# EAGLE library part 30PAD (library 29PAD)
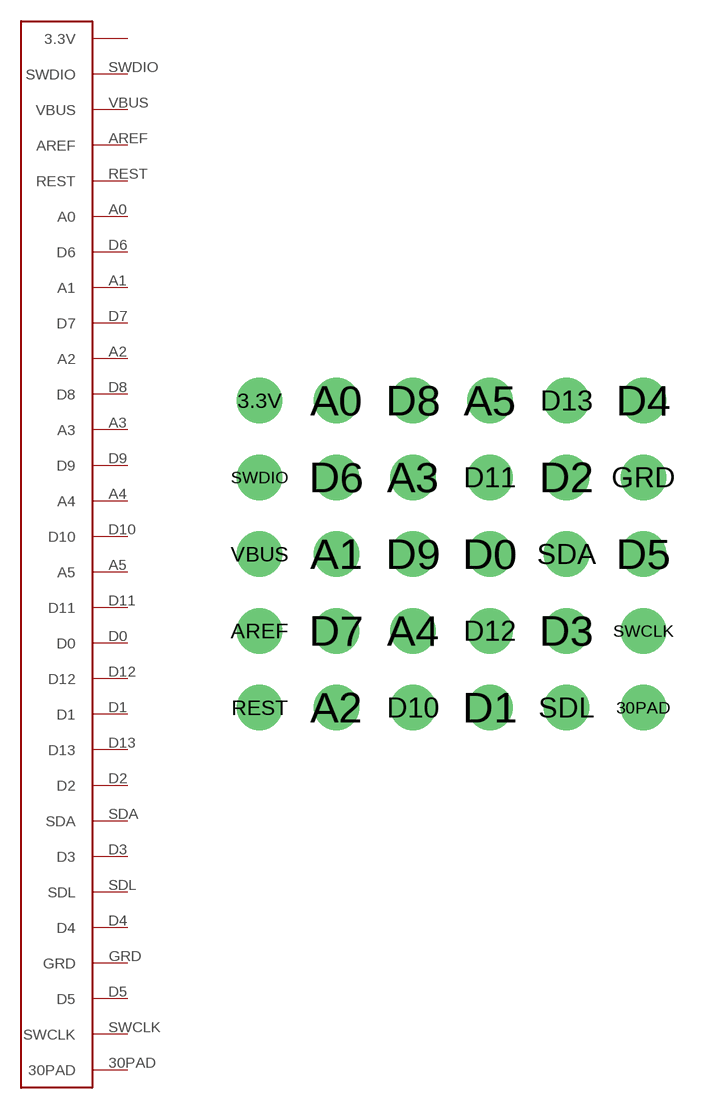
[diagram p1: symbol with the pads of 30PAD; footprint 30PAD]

Designator prefix -

## 30PAD  [30PAD]
3.3V  3.3V
30PAD  30PAD  nc
A0  A0
A1  A1
A2  A2
A3  A3
A4  A4
A5  A5
AREF  AREF
D0  D0
D1  D1
D2  D2
D3  D3
D4  D4
D5  D5
D6  D6
D7  D7
D8  D8
D9  D9
D10  D10
D11  D11
D12  D12
D13  D13
GRD  GRD
REST  REST
SDA  SDA
SDL  SDL
SWCLK  SWCLK
SWDIO  SWDIO
VBUS  VBUS

## Footprint 30PAD (pad centres in mm)
drill 1 pad 1.4: 3.3V -6.35,12.16; 30PAD 6.35,2; A0 -3.81,12.16; A1 -3.81,7.08; A2 -3.81,2; A3 -1.27,9.62; A4 -1.27,4.54; A5 1.27,12.16; AREF -6.35,4.54; D0 1.27,7.08; D1 1.27,2; D2 3.81,9.62; D3 3.81,4.54; D4 6.35,12.16; D5 6.35,7.08; D6 -3.81,9.62; D7 -3.81,4.54; D8 -1.27,12.16; D9 -1.27,7.08; D10 -1.27,2; D11 1.27,9.62; D12 1.27,4.54; D13 3.81,12.16; GRD 6.35,9.62; REST -6.35,2; SDA 3.81,7.08; SDL 3.81,2; SWCLK 6.35,4.54; SWDIO -6.35,9.62; VBUS -6.35,7.08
